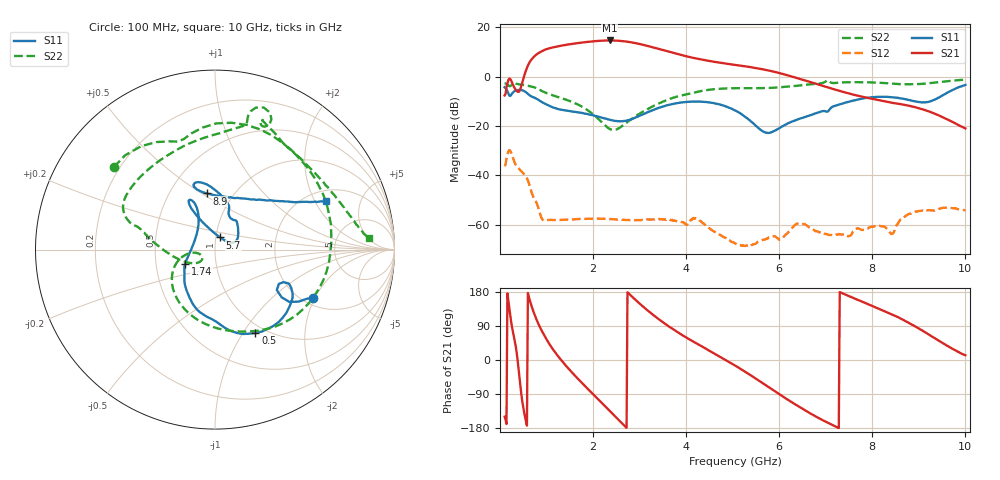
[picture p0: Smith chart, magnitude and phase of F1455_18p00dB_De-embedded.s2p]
! Integrated Device Technology
! Corporate Headquarters
! 6024 Silver Creek Valley Road
! San Jose, CA 95138  USA
! Phone:  1-408-284-8200
! Toll Free:  1-800-223-1366
! Webpage:  http://www.idt.com/
! Timing and RF Division
! 515 Groton Road, Suite 102
! Westford, MA 01886-6024
! Device:  F1455
! Description: 6-bit 0.5 dB Transmit Variable Gain Amplifier
! Frequency:  1400.0 -  2300.00 MHz
! Package:  6x6 mm Thin QFN Plastic Package: 28 pin
! State:  36
! Atten State:  18.0 dB
! Voltage:  +5.00 Volts
! Current:  217.632 mA
! Data:  The device was measured on a the F1455 evaluation board which has
!  individual transmission lines to the RF pins.  Data was collected
!  using a calibrated network analyzer.  The evaluation board was
!  de-embedded using a TRL calibration technique.
!  The reference plane is the edge of the package pin.
!  Pin  1 = CSb
!  Pin  2 = DATA
!  Pin  3 = CLK
!  Pin  4 = RSET
!  Pin  5 = GND
!  Pin  6 = RFIN  = Port 1
!  Pin  7 = GND
!  Pin  8 = NC
!  Pin  9 = NC
!  Pin 10 = NC
!  Pin 11 = NC
!  Pin 12 = NC
!  Pin 13 = NC
!  Pin 14 = /STBY
!  Pin 15 = GND
!  Pin 16 = RFOUT  = Port 2
!  Pin 17 = GND
!  Pin 18 = NC
!  Pin 19 = NC
!  Pin 20 = NC
!  Pin 21 = GND
!  Pin 22 = NC
!  Pin 23 = GND
!  Pin 24 = NC
!  Pin 25 = NC
!  Pin 26 = NC
!  Pin 27 = GND
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# GHz S dB R 50
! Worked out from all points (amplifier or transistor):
!   496 points, 100 MHz to 10 GHz, reference 50 ohm
!   highest |S21| = 14.6 dB at 2.36 GHz (marker M1)
!   |S21| within 3 dB of that: 1.096 GHz to 3.332 GHz (2.236 GHz wide, 101 % of centre)
!   unconditionally stable (mu >= 1): start of sweep to end of sweep
!   at 1.74 GHz: K = 71.54, MAG = 14.1 dB, |S12| = -57.7 dB
!   at 5.06 GHz: K = 451.27, MAG = 6.7 dB, |S12| = -67.7 dB
!   at 10 GHz: K = 399.02, MAG = -12.4 dB, |S12| = -54.2 dB
!   S11 on the Smith chart (normalised r, x): 100 MHz: 2.26, -1.92; 500 MHz: 0.90, -1.14; 1.74 GHz: 0.71, -0.11; 5.7 GHz: 1.05, +0.14; 8.9 GHz: 0.76, +0.53; 10 GHz: 2.47, +2.48
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0.1  -4.34 -26.3  -7.68 -149.6  -36.35 46.4  -2.77 140.7
0.26  -6.89 -24.7  -2.51 86.5  -31.94 -76.5  -3.30 95.7
0.38  -5.49 -41.6  -6.18 -1.2  -36.81 -116.7  -3.06 57.7
0.5  -5.75 -64.1  -1.10 -125.0  -39.22 -154.9  -3.40 26.7
0.68  -8.10 -91.0  6.96 141.8  -46.97 140.9  -4.05 -15.6
0.82  -9.39 -109.2  9.40 96.9  -52.96 116.3  -5.05 -47.0
0.96  -10.98 -123.2  10.80 63.3  -58.50 124.9  -6.39 -72.4
1.32  -13.49 -143.5  12.52 -0.8  -58.15 94.2  -8.76 -120.1
1.74  -14.70 -154.8  13.71 -57.8  -57.70 60.1  -11.99 -155.7
1.76  -14.75 -155.4  13.76 -60.3  -57.61 58.7  -12.19 -157.0
2.06  -15.99 -164.1  14.37 -97.6  -57.54 41.1  -16.26 -171.1
2.36  -17.55 179.4  14.62 -134.8  -57.82 27.8  -21.28 -161.4
2.76  -17.71 143.2  14.05 176.3  -58.16 15.8  -18.15 -143.3
3.08  -15.26 122.2  12.84 140.4  -58.27 7.9  -14.16 -162.0
3.4  -12.77 114.5  11.27 108.8  -57.77 -2.2  -11.06 -178.7
4.08  -10.22 116.1  7.86 53.8  -58.72 -14.5  -6.94 163.5
5.06  -13.81 117.6  4.70 -15.2  -67.74 -44.4  -4.73 148.0
5.7  -22.65 67.1  2.73 -65.5  -66.02 -16.1  -4.67 121.9
6.7  -15.51 39.8  -2.40 -143.2  -61.68 -127.6  -3.12 78.4
8.36  -8.29 107.6  -10.45 123.4  -62.80 123.5  -2.78 62.2
8.9  -10.01 98.2  -12.34 90.3  -54.93 129.8  -3.13 40.6
10  -3.40 23.8  -21.04 12.5  -54.19 51.4  -1.28 4.4
